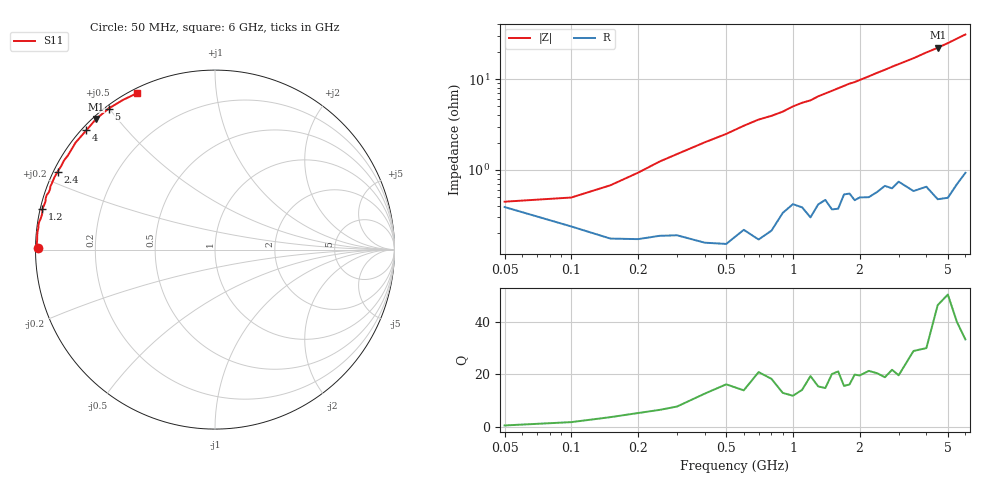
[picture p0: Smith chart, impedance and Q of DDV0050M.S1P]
! Infineon Technologies  Discrete & RF Semiconductors
! BBY58-02W
! Si Tuning Diode in SCD-80
! VR =
! S-Parameters:  June  2000
# GHz  S  MA  R  50
!  f  S11
! GHz  MAG  ANG
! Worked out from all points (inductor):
!   34 points, 50 MHz to 6 GHz, reference 50 ohm
!   read as one part to ground: L = 729 pH near 150 MHz
!   highest Q = 46.4 at 4.5 GHz (marker M1), where L = 782 pH
!   S11 on the Smith chart (normalised r, x): 50 MHz: 0.01, +0.00; 1.2 GHz: 0.01, +0.12; 2.4 GHz: 0.01, +0.23; 4 GHz: 0.01, +0.39; 5 GHz: 0.01, +0.50; 6 GHz: 0.02, +0.62
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0.05  0.9845 179.5
0.1  0.9905 179.0
0.2  0.9931 177.9
0.5  0.9939 174.3
0.7  0.9932 171.8
0.8  0.9915 171.0
0.9  0.9867 170.0
1  0.9835 168.6
1.1  0.9848 167.5
1.2  0.9882 166.7
1.3  0.9837 165.3
1.4  0.9818 164.2
1.5  0.9857 163.1
1.6  0.9855 162.0
1.7  0.9793 160.9
1.8  0.9789 159.8
1.9  0.9822 159.0
2.2  0.981 155.8
2.4  0.9785 153.6
2.6  0.9752 151.6
2.8  0.9769 149.4
3  0.973 147.4
3.5  0.9792 142.5
4  0.9776 137.1
4.5  0.9842 132.3
5  0.9843 127.0
5.5  0.9789 121.6
6  0.9735 116.4
